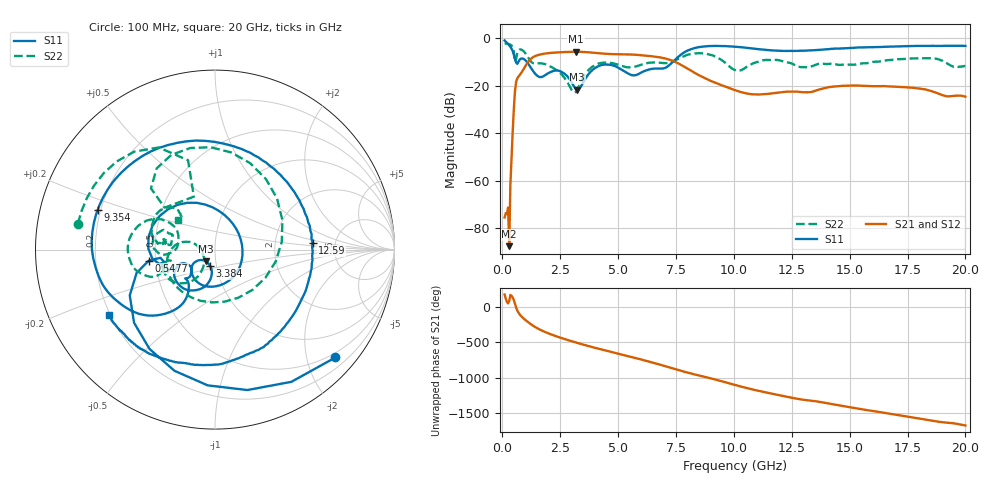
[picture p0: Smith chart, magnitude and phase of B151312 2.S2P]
!  2-Port S-parameters saved by WinCal
! VAR MeasName=S-Parameters (CALIBRATED_DATA) read from VNA (N5244A)
! VAR MeasDate=12/8/2015 5:43:58 PM
! VAR NAME=B151312 2
! VAR FILENAME=B151312 2.S2P
! VAR DATE=12/8/2015 5:43:58 PM
! VAR PHYS_PORTS=1,2
# Hz S DB R 50
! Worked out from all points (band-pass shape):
!   401 points, 100 MHz to 20 GHz, reference 50 ohm
!   highest |S21| = -5.64 dB at 3.184 GHz (marker M1); lowest = -87.4 dB at 299 MHz (marker M2)
!   |S21| within 3 dB of the highest: 1.233 GHz to 7.09 GHz (5.856 GHz wide, 141 % of centre)
!   lowest |S11| = -21.6 dB at 3.234 GHz (marker M3), VSWR 1.18, Z = 44.8 - j5.95 ohm
!   |S11| at or under -10 dB: 590 MHz to 689.5 MHz (99.42 MHz wide, 15.5 % of centre); 1.065 GHz to 7.358 GHz (6.293 GHz wide, 149 % of centre)
!   |S22| runs from -22.8 to -2.2 dB; largest |S21 - S12| = 0.0021
!   S11 on the Smith chart (normalised r, x): 100 MHz: 0.40, -2.56; 547.8 MHz: 0.46, -0.06; 3.384 GHz: 0.93, -0.17; 9.354 GHz: 0.19, +0.16; 12.59 GHz: 3.35, +0.36; 20 GHz: 0.20, -0.27
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1e8  -0.91 -41.8  -75.39 174.4  -78.39 149.1  -2.19 169.3
2.99e8  -2.95 -108.5  -87.45 82.1  -82.58 -162.6  -2.48 145.5
5.4775e8  -8.56 -170.6  -22.20 46.2  -22.20 46.2  -9.96 111.8
8.96e8  -8.57 159.2  -13.35 -156.0  -13.35 -156.0  -5.21 80.5
1.14475e9  -11.06 111.3  -9.56 137.6  -9.56 137.5  -8.53 6.7
1.44325e9  -15.15 55.3  -7.37 71.5  -7.38 71.5  -10.61 -93.5
1.9905e9  -14.65 -59.2  -6.25 -13.4  -6.24 -13.4  -11.44 -170.6
2.5875e9  -14.29 -129.5  -5.83 -82.4  -5.83 -82.4  -15.47 164.9
3.1845e9  -21.33 -134.5  -5.64 -142.3  -5.64 -142.3  -22.41 -143.4
3.23425e9  -21.61 -127.5  -5.65 -147.2  -5.65 -147.2  -21.56 -136.0
3.3835e9  -20.47 -106.7  -5.69 -161.4  -5.68 -161.4  -18.48 -123.6
3.43325e9  -19.65 -102.3  -5.71 -166.1  -5.71 -166.1  -17.47 -122.7
4.72675e9  -11.29 -145.6  -6.65 84.0  -6.64 83.9  -10.40 -161.6
5.72175e9  -15.54 -142.7  -6.91 1.6  -6.91 1.7  -11.93 -157.5
6.7665e9  -12.72 -134.7  -7.96 -90.3  -7.97 -90.4  -10.26 -163.5
8.01025e9  -5.12 -139.8  -12.79 152.4  -12.78 152.2  -6.91 -164.8
9.3535e9  -3.22 161.5  -19.31 42.0  -19.29 41.8  -8.44 153.4
1.005e10  -3.54 132.1  -21.82 -21.7  -21.85 -21.9  -13.37 161.8
1.258725e10  -5.28 4.0  -22.40 152.9  -22.40 153.6  -11.00 160.1
1.338325e10  -5.06 -32.1  -22.50 115.2  -22.44 115.6  -11.78 174.4
1.67165e10  -3.53 -111.4  -20.26 -66.2  -20.08 -66.4  -9.15 170.3
2e10  -3.19 -148.4  -24.56 127.6  -24.58 126.4  -11.67 141.5
